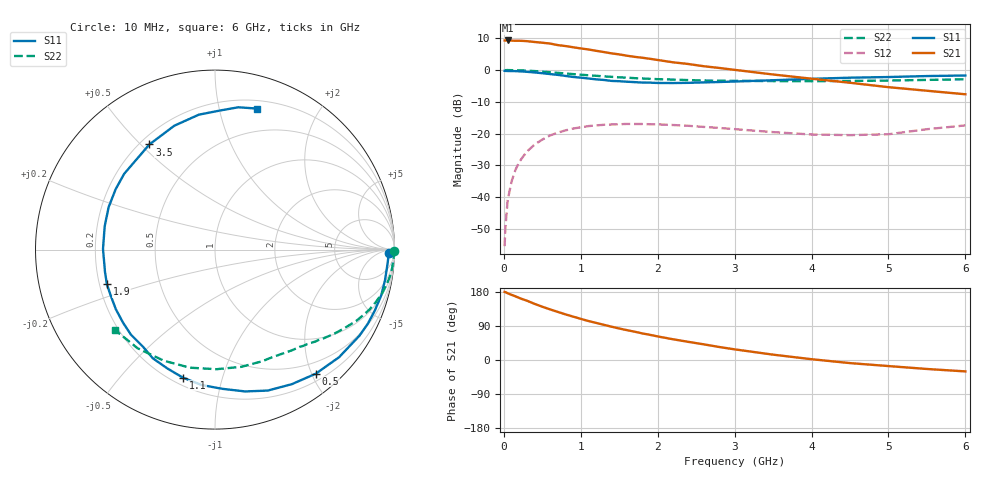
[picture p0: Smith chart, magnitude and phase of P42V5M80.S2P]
! SIEMENS Small Signal Semiconductors
! BFP182
! Si NPN RF Bipolar Junction Transistor in SOT143
! VCE = 2.5 V  IC = 0.8 mA
! Common Emitter S-Parameters:  March  1996
# GHz  S  MA  R  50
!  f  S11  S21  S12  S22
! GHz  MAG  ANG  MAG  ANG  MAG  ANG  MAG  ANG
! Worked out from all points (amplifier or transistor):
!   36 points, 10 MHz to 6 GHz, reference 50 ohm
!   highest |S21| = 9.3 dB at 50 MHz (marker M1)
!   |S21| within 3 dB of that: start of sweep to 1.14 GHz
!   unconditionally stable (mu >= 1): 2.747 GHz to end of sweep
!   at 250 MHz: K = 0.09, MSG = 18.2 dB, |S12| = -27.2 dB
!   at 1.4 GHz: K = 0.52, MSG = 11.2 dB, |S12| = -17.1 dB
!   at 6 GHz: K = 1.11, MAG = 2.9 dB, |S12| = -17.4 dB
!   S11 on the Smith chart (normalised r, x): 10 MHz: 50, -29; 500 MHz: 0.31, -2.06; 1.1 GHz: 0.24, -0.75; 1.9 GHz: 0.23, -0.15; 3.5 GHz: 0.24, +0.53; 6 GHz: 0.27, +1.30
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0.01  0.9705 -1.0  2.909 179.6  0.0017 85.9  0.9991 -0.3
0.02  0.9674 -2.0  2.913 179.1  0.0033 85.1  0.9933 -0.7
0.05  0.9642 -5.1  2.914 176.1  0.009 87.8  0.9978 -1.9
0.1  0.9625 -10.2  2.898 172.0  0.0176 82.6  0.9938 -3.8
0.2  0.9531 -20.9  2.886 163.8  0.0358 76.8  0.9892 -7.6
0.3  0.9369 -30.8  2.84 156.5  0.0522 70.1  0.9758 -11.3
0.4  0.9151 -40.9  2.758 148.1  0.0672 64.6  0.9622 -14.7
0.5  0.8908 -50.9  2.684 140.6  0.0806 58.3  0.9426 -18.1
0.6  0.8633 -60.3  2.606 133.6  0.0933 52.5  0.9233 -21.2
0.8  0.8079 -78.0  2.381 120.5  0.1123 42.6  0.8827 -26.6
1.1  0.7354 -104.1  2.104 102.8  0.1313 29.6  0.8263 -33.4
1.3  0.6976 -119.8  1.916 92.9  0.1376 22.3  0.7949 -37.4
1.5  0.6665 -134.6  1.76 83.1  0.1403 16.2  0.7667 -41.0
1.9  0.6326 -162.2  1.5 66.4  0.1405 6.2  0.727 -47.6
2.2  0.624 179.6  1.321 54.7  0.1365 0.6  0.7067 -52.5
2.8  0.6477 148.7  1.077 34.3  0.1228 -6.7  0.6777 -63.1
3.5  0.6905 122.0  0.85 14.1  0.1056 -8.6  0.6694 -77.4
4  0.7265 108.2  0.73 2.1  0.0968 -3.8  0.6664 -89.3
4.5  0.7572 96.8  0.63 -8.2  0.0946 2.2  0.6726 -102.0
5  0.7752 88.0  0.537 -16.0  0.0977 12.3  0.6817 -114.8
5.5  0.8035 80.7  0.472 -23.7  0.1173 15.3  0.6987 -128.2
6  0.8192 73.6  0.415 -30.1  0.1346 14.8  0.7143 -141.0
